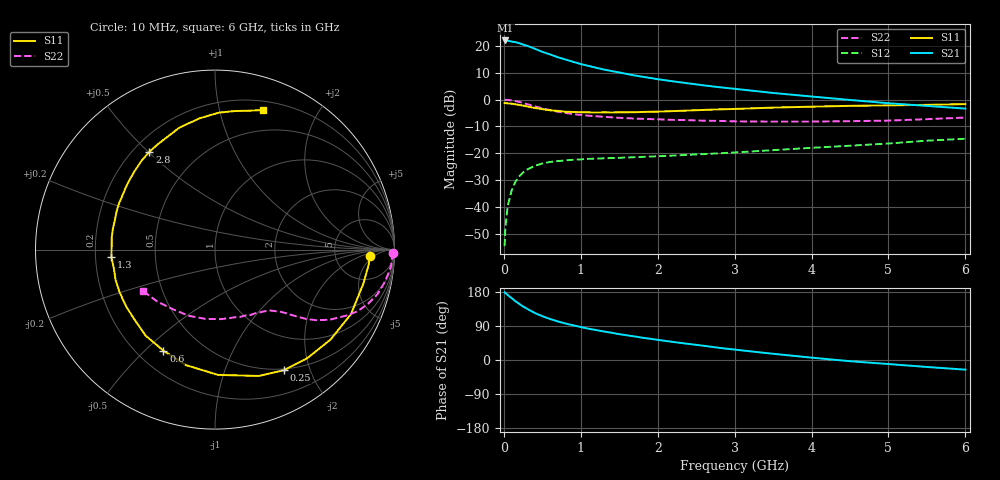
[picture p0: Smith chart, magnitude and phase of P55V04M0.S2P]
! SIEMENS Small Signal Semiconductors
! BFP183
! Si NPN RF Bipolar Junction Transistor in SOT143
! VCE = 5 V  IC = 4 mA
! Common Emitter S-Parameters:  March  1996
# GHz  S  MA  R  50
!  f  S11  S21  S12  S22
! GHz  MAG  ANG  MAG  ANG  MAG  ANG  MAG  ANG
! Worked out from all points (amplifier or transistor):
!   36 points, 10 MHz to 6 GHz, reference 50 ohm
!   highest |S21| = 21.9 dB at 20 MHz (marker M1)
!   |S21| within 3 dB of that: start of sweep to 394.9 MHz
!   unconditionally stable (mu >= 1): 1.696 GHz to 5.749 GHz
!   at 250 MHz: K = 0.18, MSG = 23.7 dB, |S12| = -27.1 dB
!   at 1.4 GHz: K = 0.86, MSG = 16.1 dB, |S12| = -21.7 dB
!   at 6 GHz: K = 0.95, MSG = 5.6 dB, |S12| = -14.5 dB
!   S11 on the Smith chart (normalised r, x): 10 MHz: 12, -4; 250 MHz: 0.48, -1.62; 600 MHz: 0.30, -0.57; 1.3 GHz: 0.27, -0.03; 2.8 GHz: 0.26, +0.50; 6 GHz: 0.28, +1.36
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0.01  0.8617 -2.5  12.32 178.4  0.0019 84.0  0.9941 -1.0
0.02  0.8609 -5.4  12.49 177.0  0.0042 87.8  0.9874 -2.1
0.05  0.8481 -12.9  12.32 171.6  0.0105 85.9  0.9851 -5.3
0.15  0.8157 -38.0  11.63 155.4  0.0297 69.2  0.9385 -15.4
0.2  0.7938 -49.6  11.11 148.1  0.0375 64.6  0.9045 -19.5
0.25  0.7739 -60.2  10.47 141.3  0.0443 59.1  0.8664 -23.3
0.3  0.7451 -70.9  9.981 135.5  0.05 54.5  0.8239 -26.4
0.4  0.6981 -88.7  8.782 124.3  0.0588 47.1  0.7497 -31.4
0.5  0.6637 -104.0  7.681 115.6  0.065 41.3  0.6876 -34.9
0.6  0.6323 -117.0  6.887 108.2  0.0694 37.6  0.6371 -37.3
0.7  0.6157 -128.9  6.102 101.9  0.072 34.2  0.5948 -39.0
0.8  0.5944 -138.8  5.539 96.3  0.0742 31.7  0.5632 -40.4
0.9  0.5879 -147.3  5.014 91.6  0.0763 30.0  0.5377 -41.5
1.1  0.579 -163.1  4.214 82.6  0.0794 27.4  0.5018 -43.6
1.3  0.5787 -175.7  3.609 75.3  0.0812 26.1  0.4776 -45.8
1.7  0.5815 163.6  2.802 62.1  0.085 25.6  0.4434 -50.7
2.2  0.6101 143.2  2.174 47.6  0.0912 26.6  0.4194 -58.0
2.8  0.6567 123.8  1.694 32.1  0.1004 27.4  0.4009 -69.1
3.5  0.7082 106.2  1.325 16.4  0.1151 28.4  0.389 -84.5
4.5  0.7635 88.3  0.982 -3.2  0.1391 26.1  0.3967 -111.8
5.5  0.7967 76.2  0.762 -18.4  0.1724 22.5  0.4325 -137.9
6  0.8227 71.0  0.679 -25.5  0.1873 18.7  0.4626 -150.1
